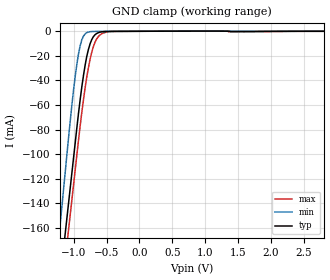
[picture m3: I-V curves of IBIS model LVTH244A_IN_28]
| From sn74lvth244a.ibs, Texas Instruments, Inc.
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[Model]   LVTH244A_IN_28
Model_type  Input
Vinl=0.8
Vinh=2.0
| variable   typ   min   max
C_comp   3.89pF   3.16pF   5.27pF
[Temperature Range]   40   -40   100
| Ambient temperature   25   -40   85
[Voltage range]   2.8   2.7   2.9
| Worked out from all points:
|   GND clamp passes 1 mA (typ) near -0.62 V on its own axis
[GND Clamp]
| LVTH244A_IN_28
|   Voltage   I(typ)   I(min)   I(max)
-5.5V     -2.408A    -2.647A    -2.409A
-1.22V    -209.4mA   -166.1mA   -230.4mA
-1.205V   -202.1mA   -157.7mA   -223.2mA
-1.125V   -163.2mA   -113.1mA   -184.6mA
-1.075V   -138.9mA   -85.4mA    -160.5mA
-975mV    -90.32mA   -36.3mA    -112.3mA
-900mV    -55.42mA   -11.62mA   -76.73mA
-800mV    -20.4mA    -1.144mA   -37.12mA
-675mV    -2.832mA   -139.6uA   -8.888mA
-575mV    -458.4uA   -111.4uA   -2.116mA
-425mV    -91.65uA   -80.03uA   -193.6uA
2.8V      16.5pA     10.34pA    -1.624nA
